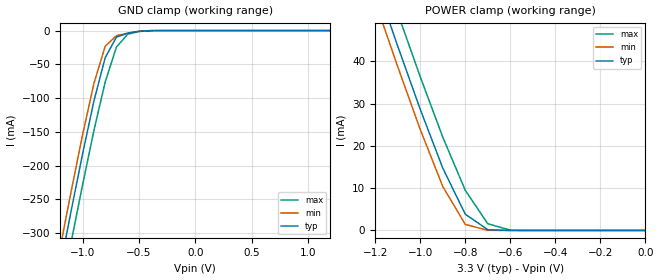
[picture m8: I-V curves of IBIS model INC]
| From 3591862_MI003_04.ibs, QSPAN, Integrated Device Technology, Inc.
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|   Model INC
[Model]   INC
Model_type   Input
Polarity   Non-Inverting
Vinl =   0.8000V
Vinh =   2.0000V
C_comp   5.00pF   5.00pF   5.00pF
[Voltage Range]   3.3000V   3.0000V   4.0000V
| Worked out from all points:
|   GND clamp passes 1 mA (typ) near -0.49 V on its own axis
|   POWER clamp passes 1 mA (typ) near -0.72 V on its own axis
[GND_clamp]
| voltage   I(typ)   I(min)   I(max)
-3.3V     -2.257A    -2.23A     -2.3A
-1.2V     -350.9mA   -322mA     -397.4mA
-1.1V     -265.2mA   -236.3mA   -311.6mA
-1V       -182.1mA   -153.8mA   -227.9mA
-900mV    -104.3mA   -78.23mA   -148mA
-800mV    -40.18mA   -23.23mA   -76.23mA
-700mV    -9.723mA   -7.586mA   -24.38mA
-600mV    -3.896mA   -3.857mA   -5.407mA
-500mV    -1.136mA   -1.021mA   -1.384mA
-400mV    -130.2uA   -83.03uA   -226.8uA
1.2V      19.95pA    4.517pA    391.4pA
[POWER_clamp]
| voltage   I(typ)   I(min)   I(max)
-3.3V     402.4mA    398mA      409.5mA
-1.2V     59mA       54.14mA    66.82mA
-1.1V     43.57mA    38.72mA    51.37mA
-1V       28.64mA    23.87mA    36.34mA
-900mV    14.76mA    10.41mA    22.07mA
-800mV    3.845mA    1.444mA    9.496mA
-700mV    187.3uA    29.52uA    1.592mA
-600mV    4.091uA    424.9nA    73.55uA
0V        43.07pA    18.3pA     650pA
